PROGRAM MAIN
VAR
	bExecute				: BOOL:=TRUE;
	sRemoteHost				: STRING(15);
	nRemotePort				: UDINT;
	asduAddr				: DWORD;
	nOrgAdd					: BYTE;

	eComState				: E_ComState	:= INIT;
	fbConnection			: FB_ClientServerConnection;
	fbProtocol				: FB_IEC870_5_104TProtocol;
	stBuffer				: ST_IEC870_5_101TBuffer;
	fbBuffer				: FB_IEC870_5_101TBufferCtrl;
	
	stTxAsdu 				: ST_IEC870_5_101AOGen; // Asdu to send 
	stRxAsdu 				: ST_IEC870_5_101AOGen; // Received asdu 
	
	tRxTimeTag				: T_CP56Time2a;			// received time tag
	
	// general interrogation
	bGenInro				: BOOL := TRUE; 		// enable general interrogation
	tGenInro				: TIME := T#20S;		// general interrogation cycle time
	nQOI_GenInro			: BYTE := INT_TO_BYTE(eIEC870_QOI_INROGEN); // qualifier of general interrogation command
	fbGenInroTimer			: TON;
	
	// counter interrogation
	bGenCountInro			: BOOL := TRUE;			// enable general counter interrogation
	tGenCountInro			: TIME := T#6S;			// general counter interrogation cycle time
	eFRZ					: E_IEC870_5_101FRZ := eIEC870_FRZ_FREEZE; // freeze counter values (default first command)
	eRQT					: E_IEC870_5_101RQT := eIEC870_RQT_REQCOGEN; // general counter group
	nQCC_GenCountInro		: BYTE := INT_TO_BYTE(eRQT) OR SHL(INT_TO_BYTE(eFRZ),6); // qualifier of counter interrogation
	fbGenCountInroTimer		: TON;
	
	// clock synchronisation
	bClockSync				: BOOL := TRUE;
	tClockSync				: TIME := T#10S;
	fbClockSyncTimer		: TON;	
	fbLocalSystemTime		: FB_LocalSystemTime;
	
	// spontaneous data transmission
	fbSpontTimer			: TON;
END_VAR

// get/refresh system time
fbLocalSystemTime(	sNetID:= '', 	//empty string - local
					bEnable:= TRUE,
					dwCycle:= 5);

// timer
fbSpontTimer(IN:= TRUE XOR fbSpontTimer.Q, PT:= T#5S);
fbGenInroTimer(IN:= bGeninro XOR fbGenInroTimer.Q, PT:= tGenInro);
fbGenCountInroTimer(IN:= bGenCountInro XOR fbGenCountInroTimer.Q, PT:= tGenCountInro);
fbClockSyncTimer(IN:= bClockSync XOR fbClockSyncTimer.Q, PT:= tClockSync);

							
// connection management
CASE eComState OF
INIT: 
	// TCP/IP connection
	sRemoteHost	:= '127.0.0.1';		// ip-address (slave)
	nRemotePort	:= 2404;			// communication port - check firewall settings
	asduAddr	:= 3;				// common asdu addr
	nOrgAdd		:= 1;				// originator addr
	
	
	// INIT protocol parameter
	fbConnection.nMode 		:= CONNECT_MODE_ENABLEDBG; 	// enable debug messages

	fbProtocol.sSrvNetID				:= '';		
	fbProtocol.protPara.sRemoteHost		:= sRemoteHost;	// slave IP-address
	fbProtocol.protPara.nRemotePort		:= nRemotePort;
	fbProtocol.protPara.bControlDT		:= TRUE;		// data transmission controlled by master - ON
	fbProtocol.protPara.bDTControlled 	:= FALSE;		// data transmission controlled by slave - OFF

	fbProtocol.protPara.bPackFrames		:= TRUE;
	fbProtocol.protPara.bThrottleMode	:= TRUE;
	fbProtocol.bOutDbg					:= FALSE;	// disable debug output


	// INIT RX/TX buffer parameter
	stBuffer.eDbg					:= eIEC870_FIFO_DBG_OFF;		// fifo debug off
	stBuffer.asduFmt.eCOTSize		:= eIEC870_COT_TwoOctets;		// cause of transfer size
	stBuffer.asduFmt.eAsduAddrSize	:= eIEC870_AsduAddr_TwoOctets;	// common asdu addr size
	stBuffer.asduFmt.eObjAddrSize	:= eIEc870_ObjAddr_ThreeOctets;	// object address size

	eComState := IDLE;
	
	
IDLE:	
	IF bExecute THEN
		stBuffer.asduSize := F_iecApdu104ToAsduLen(fbProtocol.protPara.APDULength);
		eComState := CONNECT;
	END_IF

	
CONNECT: ;
	fbConnection( 	bEnable := bExecute,
					sRemoteHost	:= fbProtocol.protPara.sRemoteHost,
					nRemotePort	:= fbProtocol.protPara.nRemotePort,
					tReconnect 	:= fbProtocol.protPara.t0 );

	CASE fbConnection.eState OF 
	eSOCKET_CONNECTED:
		fbProtocol.INIT( 	hSocket := fbConnection.hSocket,
							buffer := stBuffer );
		eComState := DATATRANSFER;			
	eSOCKET_DISCONNECTED:
		eComState := IDLE;	
	eSOCKET_SUSPENDED:
		; // wait for connection	
	END_CASE		
		

DATATRANSFER: ;
	IF bExecute THEN
		fbProtocol(buffer := stBuffer);
		IF NOT fbProtocol.bError THEN
			IF fbProtocol.eDTState = eIEC870_STARTDT THEN
				;// exchange data
			END_IF
		ELSE // error occured - log error msg. and close socket
			ADSLOGSTR(	ADSLOG_MSGTYPE_ERROR OR ADSLOG_MSGTYPE_LOG,		// log errors
						'IEC60870-5-104 Transport Interface error: %s',
						DWORD_TO_HEXSTR(fbProtocol.nErrID,0,TRUE));
			eComState := CLOSESOCKET;
		END_IF
	ELSE // stop data transfer
		fbProtocol.STOPDT(buffer := stBuffer);
		eComState := STOPDATATRANSFER;
	END_IF

	
STOPDATATRANSFER: 
	fbProtocol(buffer := stBuffer);
	IF fbProtocol.eDTState = eIEC870_STOPDT THEN
		eComState := CLOSESOCKET;	// close connection
	END_IF


CLOSESOCKET: ;
	fbConnection(bEnable := FALSE);
	IF fbConnection.eState = eSOCKET_DISCONNECTED THEN
		eComState := IDLE;
	END_IF
END_CASE


// -----------------------------------------------------------------------------------
// process received data

REPEAT
	fbBuffer.RxRemoveObj(	getObj => stRxAsdu,
 							buffer := stBuffer);
								
	IF fbBuffer.bOk THEN
		CASE stRxAsdu.ident.eType OF
		M_SP_NA_1:	// single point without time tag
			CASE stRxAsdu.info.objAddr OF 	
			10: // bSlaveToMaster
				F_iecMoveStreamToBuffer (ADR(nSIQ_bSlaveToMaster),SIZEOF(nSIQ_bSlaveToMaster), stRxAsdu.info.stream); //Copy value to local varialbe
							
				bSlaveToMaster		:= nSIQ_bSlaveToMaster.0;
				eSPI_bSlaveToMaster	:= BOOL_TO_INT(nSIQ_bSlaveToMaster.0);
				nQDS_bSlaveToMaster 	:= SHR((nSIQ_bSlaveToMaster AND 2#1111_0000),4);
			
			ELSE 
				// code for invalid object address
				EXIT; 
			END_CASE
			
		M_BO_NA_1,	// bitstring (32Bit) without time stamp (received as general interrogation data)
		M_BO_TB_1:	// bitstring (32Bit) with CP56Time2a time stamp (received as spontaneous data)
			CASE stRxAsdu.info.objAddr OF 	
			11: // nBitstring
				F_iecMoveStreamToBuffer (ADR(nBitstring),SIZEOF(nBitstring), stRxAsdu.info.stream); //Copy value to local varialbe
				F_iecMoveStreamToBuffer (ADR(nQDS_nBitstring),SIZEOF(nQDS_nBitstring), stRxAsdu.info.stream);
				IF stRxAsdu.ident.eType = M_BO_TB_1 THEN
					F_iecMoveStreamToBuffer (ADR(tRxTimeTag),SIZEOF(tRxTimeTag), stRxAsdu.info.stream);
				END_IF		
			ELSE 
				// code for invalid object address
				EXIT; 
			END_CASE
		
		M_ME_NB_1:	// measured value (scaled)
			CASE stRxAsdu.info.objAddr OF 	
			12: // nMeasurementValue
				F_iecMoveStreamToBuffer (ADR(nMeasurementValue),SIZEOF(nMeasurementValue), stRxAsdu.info.stream); //Copy value to local varialbe
				F_iecMoveStreamToBuffer (ADR(nQDS_nMeasurementValue),SIZEOF(nQDS_nMeasurementValue), stRxAsdu.info.stream);			
			ELSE 
				// code for invalid object address
				EXIT; 
			END_CASE
		
		M_ME_NC_1:	// measured value (floating point)
			CASE stRxAsdu.info.objAddr OF 	
			13: // fMeasurementValue
				F_iecMoveStreamToBuffer (ADR(fMeasurementValue),SIZEOF(fMeasurementValue), stRxAsdu.info.stream); //Copy value to local varialbe
				F_iecMoveStreamToBuffer (ADR(nQDS_fMeasurementValue),SIZEOF(nQDS_fMeasurementValue), stRxAsdu.info.stream);	
			ELSE 
				// code for invalid object address
				EXIT; 
			END_CASE
		
		M_IT_NA_1: // integrated total
			CASE stRxAsdu.info.objAddr OF
			200: // nCounter
				F_iecMoveStreamToBuffer (ADR(nBCR_nCounter),SIZEOF(nBCR_nCounter), stRxAsdu.info.stream); //Copy value to local varialbe
				F_iecMoveStreamToBuffer (ADR(nBCR_QDS),SIZEOF(nBCR_QDS), stRxAsdu.info.stream);	
			ELSE
				// code for invalid object address
				EXIT; 
			END_CASE
			
		ELSE
			// code for invalid asdu types
			EXIT;
		END_CASE
	END_IF

UNTIL NOT fbBuffer.bOk // RX fifo is empty
END_REPEAT


// -----------------------------------------------------------------------------------
// send data

IF fbProtocol.eDTState = eIEC870_STARTDT THEN

	// start general interrogation
	IF fbGenInroTimer.Q THEN

		// create asdu
		stTxAsdu.ident.eType	:= C_IC_NA_1;	// interrogation command
		stTxAsdu.info.objAddr	:= 0;			// object address
		stTxAsdu.ident.asduAddr	:= asduAddr;	// common ASDU address
		stTxAsdu.ident.bSQ		:= FALSE;		// sequence - always false
		stTxAsdu.ident.nObj		:= 1;			// number of objects
		stTxAsdu.ident.eCOT		:= eIEC870_COT_ACT;	// cause of transmission - command activation
		stTxAsdu.ident.nORG		:= nOrgAdd;		// originator address
		stTxAsdu.ident.bPN		:= FALSE;		// positive/negative confirmation flag
		stTxAsdu.ident.bT		:= FALSE;		// test flag - not used
		stTxAsdu.ident.eClass	:= eIEC870_Class_1; // priority class

		F_iecResetStream(0,stTxAsdu.info.stream);
		F_iecCopyBufferToStream(ADR(nQOI_GenInro),SIZEOF(nQOI_GenInro), stTxAsdu.info.stream);	// copy values to transmit stream	
		fbBuffer.TxAddObj(	putObj := stTxAsdu,
							buffer := stBuffer);
				
		IF NOT fbBuffer.bOk THEN
			// code for buffer overflow
			RETURN; 
		END_IF
	END_IF

	
	// start general counter interrogation
	IF fbGenCountInroTimer.Q THEN

		// set qualifier of counter interrogation
		eRQT := eIEC870_RQT_REQCOGEN; // set general counter group
		nQCC_GenCountInro := INT_TO_BYTE(eRQT) OR SHL(INT_TO_BYTE(eFRZ),6);

		// first counter interrogation command performs freeze of counter values
		// next counter interrogation command reads counter values
		IF eFRZ = eIEC870_FRZ_FREEZE THEN
			eFRZ := eIEC870_FRZ_READ; // set next command to read counter values
		ELSE
			eFRZ := eIEC870_FRZ_FREEZE; // set next command to freeze counter values
		END_IF 
	
		// create asdu
		stTxAsdu.ident.eType	:= C_CI_NA_1;		// counter interrogation command
		stTxAsdu.info.objAddr	:= 0;				// object address
		stTxAsdu.ident.asduAddr	:= asduAddr;		// common ASDU address
		stTxAsdu.ident.bSQ		:= FALSE;			// sequence - always false
		stTxAsdu.ident.nObj		:= 1;				// number of objects
		stTxAsdu.ident.eCOT		:= eIEC870_COT_ACT;	// cause of transmission - command activation
		stTxAsdu.ident.nORG		:= nOrgAdd;			// originator address
		stTxAsdu.ident.bPN		:= FALSE;			// positive/negative confirmation flag
		stTxAsdu.ident.bT		:= FALSE;			// test flag - not used
		stTxAsdu.ident.eClass	:= eIEC870_Class_1; // priority class
		
	
		F_iecResetStream(0,stTxAsdu.info.stream);
		F_iecCopyBufferToStream(ADR(nQCC_GenCountInro),SIZEOF(nQCC_GenCountInro), stTxAsdu.info.stream);	// copy values TO transmit stream	
		fbBuffer.TxAddObj(	putObj := stTxAsdu,
							buffer := stBuffer);							
		IF NOT fbBuffer.bOk THEN
			// code for buffer overflow
			RETURN; 
		END_IF
	END_IF
	
	
	// start clock synchronisation 
	IF fbClockSyncTimer.Q AND_THEN fbLocalSystemTime.bValid THEN
	
		// create CP56Time2a timestruct
		IF fbLocalSystemTime.tzID = eTimeZoneID_Daylight THEN
			bDSTime := TRUE;
		ELSE
			bDSTime := FALSE;	
		END_IF
	
		tActTime := SYSTEMTIME_TO_CP56Time2a(fbLocalSystemTime.systemTime, bDSTime);

		// create asdu
		stTxAsdu.ident.eType	:= C_CS_NA_1;		// clock syncronisation command
		stTxAsdu.info.objAddr	:= 0;				// object address
		stTxAsdu.ident.asduAddr	:= asduAddr;		// common ASDU address
		stTxAsdu.ident.bSQ		:= FALSE;			// sequence - always false
		stTxAsdu.ident.nObj		:= 1;				// number of objects
		stTxAsdu.ident.eCOT		:= eIEC870_COT_ACT;	// cause of transmission - command activation
		stTxAsdu.ident.nORG		:= nOrgAdd;			// originator address
		stTxAsdu.ident.bPN		:= FALSE;			// positive/negative confirmation flag
		stTxAsdu.ident.bT		:= FALSE;			// test flag - not used
		stTxAsdu.ident.eClass	:= eIEC870_Class_1; // priority class

		F_iecResetStream(0,stTxAsdu.info.stream);
		F_iecCopyBufferToStream(ADR(tActTime), 7(*Please don't use the SIZEOF operator! SIZEOF returns 8 byte size for the T_CP56Time2a type (1 additional alignment byte).*), stTxAsdu.info.stream);	// copy values TO transmit stream	
		fbBuffer.TxAddObj(	putObj := stTxAsdu,
							buffer := stBuffer);
				
		IF NOT fbBuffer.bOk THEN
			// code for buffer overflow
			RETURN; 
		END_IF
	END_IF
	
	
	// send command on timer expiration or when command data value changes
	IF fbSpontTimer.Q OR_ELSE (nSCO_bMasterToSlave.0 <> bMasterToSlave) THEN
	// send single commmands - C_SC_NA_1
	
		//bMasterToSlave	
		nSCO_bMasterToSlave.0	:= bMasterToSlave;
		eSCS_bMasterToSlave		:= BOOL_TO_INT(bMasterToSlave);
		nSCO_bMasterToSlave		:= nSCO_bMasterToSlave OR SHL(INT_TO_BYTE(eQU_bMasterToSlave),2);
		nSCO_bMasterToSlave.7	:= 0;// set S/E bit (0 -> Select command, 1 -> Execute command)
	
		// create asdu - bMasterToSlave
		stTxAsdu.ident.eType	:= C_SC_NA_1;		// single command without time tag
		stTxAsdu.info.objAddr	:= 101;				// objecct address
		stTxAsdu.ident.asduAddr	:= asduAddr;		// common ASDU address
		stTxAsdu.ident.bSQ		:= FALSE;			// sequence - always false
		stTxAsdu.ident.nObj		:= 1;				// number of objects
		stTxAsdu.ident.eCOT		:= eIEC870_COT_ACT;	// cause of transmission - spontaneous
		stTxAsdu.ident.nORG		:= nOrgAdd;			// originator address
		stTxAsdu.ident.bPN		:= FALSE;			// positive/negative confirmation flag
		stTxAsdu.ident.bT		:= FALSE;			// test flag - not used
		stTxAsdu.ident.eClass	:= eIEC870_Class_1; // priority class
		
		F_iecResetStream(0,stTxAsdu.info.stream);
		F_iecCopyBufferToStream(ADR(nSCO_bMasterToSlave),SIZEOF(nSCO_bMasterToSlave), stTxAsdu.info.stream);		
		fbBuffer.TxAddObj(	putObj := stTxAsdu,
							buffer := stBuffer);
							
		IF NOT fbBuffer.bOk THEN
			// code for buffer overflow
			RETURN; 
		END_IF						
	
	END_IF	
END_IF

END_PROGRAM
